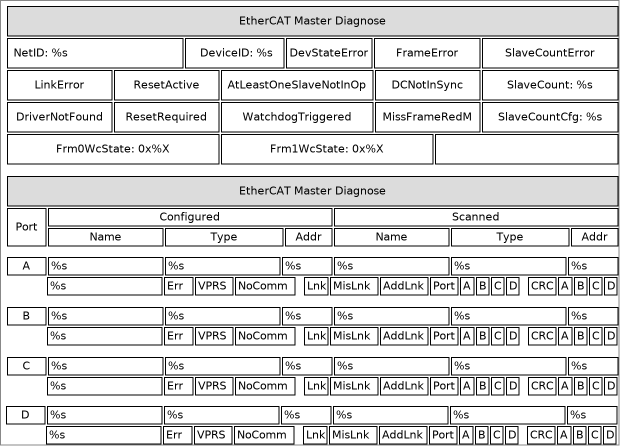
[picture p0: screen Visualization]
VISUALIZATION Visualization  // 620x446
    Rectangle (7,6 611x30), "EtherCAT Master Diagnose"
    Rectangle (7,38 176x30), "NetID: %s", text variable: MAIN.sEcMasterNetId
    Rectangle (185,38 99x30), "DeviceID: %s", text variable: MAIN.nEcMasterDeviceId
    Rectangle (286,38 86x30), "DevStateError", colour toggle: MAIN.bMasterDevStateError
    Rectangle (374,38 106x30), "FrameError", colour toggle: MAIN.bFrameWcStateError
    Rectangle (482,38 136x30), "SlaveCountError", colour toggle: MAIN.bSlaveCountError
    Rectangle (7,70 105x30), "LinkError", colour toggle: MAIN.stMasterDevState.bLinkError
    Rectangle (114,70 105x30), "ResetActive", colour toggle: MAIN.stMasterDevState.bResetActive
    Rectangle (114,102 105x30), "ResetRequired", colour toggle: MAIN.stMasterDevState.bResetRequired
    Rectangle (7,102 105x30), "DriverNotFound", colour toggle: MAIN.stMasterDevState.bDriverNotFound
    Rectangle (221,70 152x30), "AtLeastOneSlaveNotInOp", colour toggle: MAIN.stMasterDevState.bAtLeastOneNotInOp
    Rectangle (221,102 152x30), "WatchdogTriggered", colour toggle: MAIN.stMasterDevState.bWatchdogTriggerd
    Rectangle (375,70 105x30), "DCNotInSync", colour toggle: MAIN.stMasterDevState.bDcNotInSync
    Rectangle (375,102 105x30), "MissFrameRedM", colour toggle: MAIN.stMasterDevState.bMissFrmRedMode
    Rectangle (482,70 136x30), "SlaveCount: %s", text variable: MAIN.nEcMasterSlaveCount, colour toggle: MAIN.bSlaveCountError
    Rectangle (482,102 136x30), "SlaveCountCfg: %s", text variable: MAIN.nEcMasterSlaveCountCfg, colour toggle: MAIN.bSlaveCountError
    Rectangle (7,134 212x30), "Frm0WcState: 0x%X", text variable: FAST.wFrmXWcState, colour toggle: NOT FAST.bFrameWcStateOK
    Rectangle (221,134 212x30), "Frm1WcState: 0x%X", text variable: MAIN.wFrmXWcState, colour toggle: NOT MAIN.bFrameWcStateOK
    Rectangle (435,134 183x30)
    Rectangle (7,176 611x30), "EtherCAT Master Diagnose"
    Rectangle (7,208 39x38), "Port"
    Rectangle (48,208 284x18), "Configured"
    Rectangle (334,208 284x18), "Scanned"
    Rectangle (48,228 115x18), "Name"
    Rectangle (165,228 118x18), "Type"
    Rectangle (285,228 47x18), "Addr"
    Rectangle (451,228 118x18), "Type"
    Rectangle (334,228 115x18), "Name"
    Rectangle (571,228 47x18), "Addr"
    Rectangle (7,257 39x18), "A", invisible if: NOT MAIN.arrDiagSlaveInfo[0].bDiagData
    Rectangle (48,257 115x18), "%s", text variable: MAIN.arrDiagSlaveInfo[0].sName, colour toggle: MAIN.arrDiagSlaveInfoScanned[0].bDifferentName, invisible if: NOT MAIN.arrDiagSlaveInfo[0].bDiagData
    Rectangle (334,257 115x18), "%s", text variable: MAIN.arrDiagSlaveInfoScanned[0].sName, colour toggle: MAIN.arrDiagSlaveInfoScanned[0].bDifferentName, invisible if: NOT MAIN.arrDiagSlaveInfo[0].bDiagData
    Rectangle (165,257 115x18), "%s", text variable: MAIN.arrDiagSlaveInfo[0].sType, colour toggle: MAIN.arrDiagSlaveInfoScanned[0].bDifferentType, invisible if: NOT MAIN.arrDiagSlaveInfo[0].bDiagData
    Rectangle (451,257 115x18), "%s", text variable: MAIN.arrDiagSlaveInfoScanned[0].sType, colour toggle: MAIN.arrDiagSlaveInfoScanned[0].bDifferentType, invisible if: NOT MAIN.arrDiagSlaveInfo[0].bDiagData
    Rectangle (282,257 50x18), "%s", text variable: MAIN.arrDiagSlaveInfo[0].nECAddr, colour toggle: MAIN.arrDiagSlaveInfoScanned[0].bDifferentAddr, invisible if: NOT MAIN.arrDiagSlaveInfo[0].bDiagData
    Rectangle (568,257 50x18), "%s", text variable: MAIN.arrDiagSlaveInfoScanned[0].nECAddr, colour toggle: MAIN.arrDiagSlaveInfoScanned[0].bDifferentAddr, invisible if: NOT MAIN.arrDiagSlaveInfo[0].bDiagData
    Rectangle (47,277 115x18), "%s", text variable: MAIN.arrDiagSlaveInfo[0].stState.eEcState, colour toggle: MAIN.arrDiagSlaveInfo[0].stState.eEcState <> 8, invisible if: NOT MAIN.arrDiagSlaveInfo[0].bDiagData
    Rectangle (164,277 29x18), "Err", colour toggle: MAIN.arrDiagSlaveInfo[0].stState.bError, invisible if: NOT MAIN.arrDiagSlaveInfo[0].bDiagData
    Rectangle (195,277 38x18), "VPRS", colour toggle: MAIN.arrDiagSlaveInfo[0].stState.bInvalidVPRS, invisible if: NOT MAIN.arrDiagSlaveInfo[0].bDiagData
    Rectangle (235,277 60x18), "NoComm", colour toggle: MAIN.arrDiagSlaveInfo[0].stState.bNoCommToSlave, invisible if: NOT MAIN.arrDiagSlaveInfo[0].bDiagData
    Rectangle (304,277 24x18), "Lnk", colour toggle: MAIN.arrDiagSlaveInfo[0].stState.bLinkError, invisible if: NOT MAIN.arrDiagSlaveInfo[0].bDiagData
    Rectangle (330,277 48x18), "MisLnk", colour toggle: MAIN.arrDiagSlaveInfo[0].stState.bMissingLink, invisible if: NOT MAIN.arrDiagSlaveInfo[0].bDiagData
    Rectangle (380,277 48x18), "AddLnk", colour toggle: MAIN.arrDiagSlaveInfo[0].stState.bUnexpectedLink, invisible if: NOT MAIN.arrDiagSlaveInfo[0].bDiagData
    Rectangle (430,277 28x18), "Port", invisible if: NOT MAIN.arrDiagSlaveInfo[0].bDiagData
    Rectangle (460,277 14x18), "A", colour toggle: MAIN.arrDiagSlaveInfo[0].stState.bPortA, invisible if: NOT MAIN.arrDiagSlaveInfo[0].bDiagData
    Rectangle (476,277 13x18), "B", colour toggle: MAIN.arrDiagSlaveInfo[0].stState.bPortB, invisible if: NOT MAIN.arrDiagSlaveInfo[0].bDiagData
    Rectangle (491,277 13x18), "C", colour toggle: MAIN.arrDiagSlaveInfo[0].stState.bPortC, invisible if: NOT MAIN.arrDiagSlaveInfo[0].bDiagData
    Rectangle (506,277 13x18), "D", colour toggle: MAIN.arrDiagSlaveInfo[0].stState.bPortD, invisible if: NOT MAIN.arrDiagSlaveInfo[0].bDiagData
    Rectangle (528,277 28x18), "CRC", colour toggle: MAIN.arrDiagSlaveInfo[0].nSumCRCErrors <> 0, invisible if: NOT MAIN.arrDiagSlaveInfo[0].bDiagData
    Rectangle (558,277 14x18), "A", colour toggle: MAIN.arrDiagSlaveInfo[0].stPortCRCErrors.portA <> 0, invisible if: NOT MAIN.arrDiagSlaveInfo[0].bDiagData
    Rectangle (574,277 13x18), "B", colour toggle: MAIN.arrDiagSlaveInfo[0].stPortCRCErrors.portB <> 0, invisible if: NOT MAIN.arrDiagSlaveInfo[0].bDiagData
    Rectangle (589,277 13x18), "C", colour toggle: MAIN.arrDiagSlaveInfo[0].stPortCRCErrors.portC <> 0, invisible if: NOT MAIN.arrDiagSlaveInfo[0].bDiagData
    Rectangle (604,277 13x18), "D", colour toggle: MAIN.arrDiagSlaveInfo[0].stPortCRCErrors.portD <> 0, invisible if: NOT MAIN.arrDiagSlaveInfo[0].bDiagData
    Rectangle (7,307 39x18), "B", invisible if: MAIN.fbEtherCATDiag.iDiagIndex[1]=0
    Rectangle (48,307 115x18), "%s", text variable: MAIN.arrDiagSlaveInfo[1].sName, colour toggle: MAIN.arrDiagSlaveInfoScanned[1].bDifferentName, invisible if: MAIN.fbEtherCATDiag.iDiagIndex[1]=0
    Rectangle (334,307 115x18), "%s", text variable: MAIN.arrDiagSlaveInfoScanned[1].sName, colour toggle: MAIN.arrDiagSlaveInfoScanned[1].bDifferentName, invisible if: MAIN.fbEtherCATDiag.iDiagIndex[1]=0
    Rectangle (165,307 115x18), "%s", text variable: MAIN.arrDiagSlaveInfo[1].sType, colour toggle: MAIN.arrDiagSlaveInfoScanned[1].bDifferentType, invisible if: MAIN.fbEtherCATDiag.iDiagIndex[1]=0
    Rectangle (451,307 115x18), "%s", text variable: MAIN.arrDiagSlaveInfoScanned[1].sType, colour toggle: MAIN.arrDiagSlaveInfoScanned[1].bDifferentType, invisible if: MAIN.fbEtherCATDiag.iDiagIndex[1]=0
    Rectangle (282,307 50x18), "%s", text variable: MAIN.arrDiagSlaveInfo[1].nECAddr, colour toggle: MAIN.arrDiagSlaveInfoScanned[1].bDifferentAddr, invisible if: MAIN.fbEtherCATDiag.iDiagIndex[1]=0
    Rectangle (568,307 50x18), "%s", text variable: MAIN.arrDiagSlaveInfoScanned[1].nECAddr, colour toggle: MAIN.arrDiagSlaveInfoScanned[1].bDifferentAddr, invisible if: MAIN.fbEtherCATDiag.iDiagIndex[1]=0
    Rectangle (47,327 115x18), "%s", text variable: MAIN.arrDiagSlaveInfo[1].stState.eEcState, colour toggle: MAIN.arrDiagSlaveInfo[1].stState.eEcState <> 8, invisible if: MAIN.fbEtherCATDiag.iDiagIndex[1]=0
    Rectangle (164,327 29x18), "Err", colour toggle: MAIN.arrDiagSlaveInfo[1].stState.bError, invisible if: MAIN.fbEtherCATDiag.iDiagIndex[1]=0
    Rectangle (195,327 38x18), "VPRS", colour toggle: MAIN.arrDiagSlaveInfo[1].stState.bInvalidVPRS, invisible if: MAIN.fbEtherCATDiag.iDiagIndex[1]=0
    Rectangle (235,327 60x18), "NoComm", colour toggle: MAIN.arrDiagSlaveInfo[1].stState.bNoCommToSlave, invisible if: MAIN.fbEtherCATDiag.iDiagIndex[1]=0
    Rectangle (304,327 24x18), "Lnk", colour toggle: MAIN.arrDiagSlaveInfo[1].stState.bLinkError, invisible if: MAIN.fbEtherCATDiag.iDiagIndex[1]=0
    Rectangle (330,327 48x18), "MisLnk", colour toggle: MAIN.arrDiagSlaveInfo[1].stState.bMissingLink, invisible if: MAIN.fbEtherCATDiag.iDiagIndex[1]=0
    Rectangle (380,327 48x18), "AddLnk", colour toggle: MAIN.arrDiagSlaveInfo[1].stState.bUnexpectedLink, invisible if: MAIN.fbEtherCATDiag.iDiagIndex[1]=0
    Rectangle (430,327 28x18), "Port", invisible if: MAIN.fbEtherCATDiag.iDiagIndex[1]=0
    Rectangle (460,327 14x18), "A", colour toggle: MAIN.arrDiagSlaveInfo[1].stState.bPortA, invisible if: MAIN.fbEtherCATDiag.iDiagIndex[1]=0
    Rectangle (476,327 13x18), "B", colour toggle: MAIN.arrDiagSlaveInfo[1].stState.bPortB, invisible if: MAIN.fbEtherCATDiag.iDiagIndex[1]=0
    Rectangle (491,327 13x18), "C", colour toggle: MAIN.arrDiagSlaveInfo[1].stState.bPortC, invisible if: MAIN.fbEtherCATDiag.iDiagIndex[1]=0
    Rectangle (506,327 13x18), "D", colour toggle: MAIN.arrDiagSlaveInfo[1].stState.bPortD, invisible if: MAIN.fbEtherCATDiag.iDiagIndex[1]=0
    Rectangle (528,327 28x18), "CRC", colour toggle: MAIN.arrDiagSlaveInfo[1].nSumCRCErrors <> 0, invisible if: MAIN.fbEtherCATDiag.iDiagIndex[1]=0
    Rectangle (558,327 14x18), "A", colour toggle: MAIN.arrDiagSlaveInfo[1].stPortCRCErrors.portA <> 0, invisible if: MAIN.fbEtherCATDiag.iDiagIndex[1]=0
    Rectangle (574,327 13x18), "B", colour toggle: MAIN.arrDiagSlaveInfo[1].stPortCRCErrors.portB <> 0, invisible if: MAIN.fbEtherCATDiag.iDiagIndex[1]=0
    Rectangle (589,327 13x18), "C", colour toggle: MAIN.arrDiagSlaveInfo[1].stPortCRCErrors.portC <> 0, invisible if: MAIN.fbEtherCATDiag.iDiagIndex[1]=0
    Rectangle (604,327 13x18), "D", colour toggle: MAIN.arrDiagSlaveInfo[1].stPortCRCErrors.portD <> 0, invisible if: MAIN.fbEtherCATDiag.iDiagIndex[1]=0
    Rectangle (7,357 39x18), "C", invisible if: MAIN.fbEtherCATDiag.iDiagIndex[2]=0
    Rectangle (48,357 115x18), "%s", text variable: MAIN.arrDiagSlaveInfo[2].sName, colour toggle: MAIN.arrDiagSlaveInfoScanned[2].bDifferentName, invisible if: MAIN.fbEtherCATDiag.iDiagIndex[2]=0
    Rectangle (334,357 115x18), "%s", text variable: MAIN.arrDiagSlaveInfo[2].sName, colour toggle: MAIN.arrDiagSlaveInfoScanned[2].bDifferentName, invisible if: MAIN.fbEtherCATDiag.iDiagIndex[2]=0
    Rectangle (165,357 115x18), "%s", text variable: MAIN.arrDiagSlaveInfo[2].sType, colour toggle: MAIN.arrDiagSlaveInfoScanned[2].bDifferentType, invisible if: MAIN.fbEtherCATDiag.iDiagIndex[2]=0
    Rectangle (451,357 115x18), "%s", text variable: MAIN.arrDiagSlaveInfoScanned[2].sType, colour toggle: MAIN.arrDiagSlaveInfoScanned[2].bDifferentType, invisible if: MAIN.fbEtherCATDiag.iDiagIndex[2]=0
    Rectangle (282,357 50x18), "%s", text variable: MAIN.arrDiagSlaveInfo[2].nECAddr, colour toggle: MAIN.arrDiagSlaveInfoScanned[2].bDifferentAddr, invisible if: MAIN.fbEtherCATDiag.iDiagIndex[2]=0
    Rectangle (568,357 50x18), "%s", text variable: MAIN.arrDiagSlaveInfoScanned[2].nECAddr, colour toggle: MAIN.arrDiagSlaveInfoScanned[2].bDifferentAddr, invisible if: MAIN.fbEtherCATDiag.iDiagIndex[2]=0
    Rectangle (47,377 115x18), "%s", text variable: MAIN.arrDiagSlaveInfo[2].stState.eEcState, colour toggle: MAIN.arrDiagSlaveInfo[2].stState.eEcState <> 8, invisible if: MAIN.fbEtherCATDiag.iDiagIndex[2]=0
    Rectangle (164,377 29x18), "Err", colour toggle: MAIN.arrDiagSlaveInfo[2].stState.bError, invisible if: MAIN.fbEtherCATDiag.iDiagIndex[2]=0
    Rectangle (195,377 38x18), "VPRS", colour toggle: MAIN.arrDiagSlaveInfo[2].stState.bInvalidVPRS, invisible if: MAIN.fbEtherCATDiag.iDiagIndex[2]=0
    Rectangle (235,377 60x18), "NoComm", colour toggle: MAIN.arrDiagSlaveInfo[2].stState.bNoCommToSlave, invisible if: MAIN.fbEtherCATDiag.iDiagIndex[2]=0
    Rectangle (304,377 24x18), "Lnk", colour toggle: MAIN.arrDiagSlaveInfo[2].stState.bLinkError, invisible if: MAIN.fbEtherCATDiag.iDiagIndex[2]=0
    Rectangle (330,377 48x18), "MisLnk", colour toggle: MAIN.arrDiagSlaveInfo[2].stState.bMissingLink, invisible if: MAIN.fbEtherCATDiag.iDiagIndex[2]=0
    Rectangle (380,377 48x18), "AddLnk", colour toggle: MAIN.arrDiagSlaveInfo[2].stState.bUnexpectedLink, invisible if: MAIN.fbEtherCATDiag.iDiagIndex[2]=0
    Rectangle (430,377 28x18), "Port", invisible if: MAIN.fbEtherCATDiag.iDiagIndex[2]=0
    Rectangle (460,377 14x18), "A", colour toggle: MAIN.arrDiagSlaveInfo[2].stState.bPortA, invisible if: MAIN.fbEtherCATDiag.iDiagIndex[2]=0
    Rectangle (476,377 13x18), "B", colour toggle: MAIN.arrDiagSlaveInfo[2].stState.bPortB, invisible if: MAIN.fbEtherCATDiag.iDiagIndex[2]=0
    Rectangle (491,377 13x18), "C", colour toggle: MAIN.arrDiagSlaveInfo[2].stState.bPortC, invisible if: MAIN.fbEtherCATDiag.iDiagIndex[2]=0
    Rectangle (506,377 13x18), "D", colour toggle: MAIN.arrDiagSlaveInfo[2].stState.bPortD, invisible if: MAIN.fbEtherCATDiag.iDiagIndex[2]=0
    Rectangle (528,377 28x18), "CRC", colour toggle: MAIN.arrDiagSlaveInfo[2].nSumCRCErrors <> 0, invisible if: MAIN.fbEtherCATDiag.iDiagIndex[2]=0
    Rectangle (558,377 14x18), "A", colour toggle: MAIN.arrDiagSlaveInfo[2].stPortCRCErrors.portA <> 0, invisible if: MAIN.fbEtherCATDiag.iDiagIndex[2]=0
    Rectangle (574,377 13x18), "B", colour toggle: MAIN.arrDiagSlaveInfo[2].stPortCRCErrors.portB <> 0, invisible if: MAIN.fbEtherCATDiag.iDiagIndex[2]=0
    Rectangle (589,377 13x18), "C", colour toggle: MAIN.arrDiagSlaveInfo[2].stPortCRCErrors.portC <> 0, invisible if: MAIN.fbEtherCATDiag.iDiagIndex[2]=0
    Rectangle (604,377 13x18), "D", colour toggle: MAIN.arrDiagSlaveInfo[2].stPortCRCErrors.portD <> 0, invisible if: MAIN.fbEtherCATDiag.iDiagIndex[2]=0
    Rectangle (6,406 39x18), "D", invisible if: MAIN.fbEtherCATDiag.iDiagIndex[3]=0
    Rectangle (47,406 115x18), "%s", text variable: MAIN.arrDiagSlaveInfo[3].sName, colour toggle: MAIN.arrDiagSlaveInfoScanned[3].bDifferentName, invisible if: MAIN.fbEtherCATDiag.iDiagIndex[3]=0
    Rectangle (333,406 115x18), "%s", text variable: MAIN.arrDiagSlaveInfoScanned[3].sName, colour toggle: MAIN.arrDiagSlaveInfoScanned[3].bDifferentName, invisible if: MAIN.fbEtherCATDiag.iDiagIndex[3]=0
    Rectangle (164,406 115x18), "%s", text variable: MAIN.arrDiagSlaveInfo[3].sType, colour toggle: MAIN.arrDiagSlaveInfoScanned[3].bDifferentType, invisible if: MAIN.fbEtherCATDiag.iDiagIndex[3]=0
    Rectangle (450,406 115x18), "%s", text variable: MAIN.arrDiagSlaveInfoScanned[3].sType, colour toggle: MAIN.arrDiagSlaveInfoScanned[3].bDifferentType, invisible if: MAIN.fbEtherCATDiag.iDiagIndex[3]=0
    Rectangle (281,406 50x18), "%s", text variable: MAIN.arrDiagSlaveInfo[3].nECAddr, colour toggle: MAIN.arrDiagSlaveInfoScanned[3].bDifferentAddr, invisible if: MAIN.fbEtherCATDiag.iDiagIndex[3]=0
    Rectangle (567,406 50x18), "%s", text variable: MAIN.arrDiagSlaveInfoScanned[3].nECAddr, colour toggle: MAIN.arrDiagSlaveInfoScanned[3].bDifferentAddr, invisible if: MAIN.fbEtherCATDiag.iDiagIndex[3]=0
    Rectangle (46,426 115x18), "%s", text variable: MAIN.arrDiagSlaveInfo[3].stState.eEcState, colour toggle: MAIN.arrDiagSlaveInfo[3].stState.eEcState <> 8, invisible if: MAIN.fbEtherCATDiag.iDiagIndex[3]=0
    Rectangle (163,426 29x18), "Err", colour toggle: MAIN.arrDiagSlaveInfo[3].stState.bError, invisible if: MAIN.fbEtherCATDiag.iDiagIndex[3]=0
    Rectangle (194,426 38x18), "VPRS", colour toggle: MAIN.arrDiagSlaveInfo[3].stState.bInvalidVPRS, invisible if: MAIN.fbEtherCATDiag.iDiagIndex[3]=0
    Rectangle (234,426 60x18), "NoComm", colour toggle: MAIN.arrDiagSlaveInfo[3].stState.bNoCommToSlave, invisible if: MAIN.fbEtherCATDiag.iDiagIndex[3]=0
    Rectangle (303,426 24x18), "Lnk", colour toggle: MAIN.arrDiagSlaveInfo[3].stState.bLinkError, invisible if: MAIN.fbEtherCATDiag.iDiagIndex[3]=0
    Rectangle (329,426 48x18), "MisLnk", colour toggle: MAIN.arrDiagSlaveInfo[3].stState.bMissingLink, invisible if: MAIN.fbEtherCATDiag.iDiagIndex[3]=0
    Rectangle (379,426 48x18), "AddLnk", colour toggle: MAIN.arrDiagSlaveInfo[3].stState.bUnexpectedLink, invisible if: MAIN.fbEtherCATDiag.iDiagIndex[3]=0
    Rectangle (429,426 28x18), "Port", invisible if: MAIN.fbEtherCATDiag.iDiagIndex[3]=0
    Rectangle (459,426 14x18), "A", colour toggle: MAIN.arrDiagSlaveInfo[3].stState.bPortA, invisible if: MAIN.fbEtherCATDiag.iDiagIndex[3]=0
    Rectangle (475,426 13x18), "B", colour toggle: MAIN.arrDiagSlaveInfo[3].stState.bPortB, invisible if: MAIN.fbEtherCATDiag.iDiagIndex[3]=0
    Rectangle (490,426 13x18), "C", colour toggle: MAIN.arrDiagSlaveInfo[3].stState.bPortC, invisible if: MAIN.fbEtherCATDiag.iDiagIndex[3]=0
    Rectangle (505,426 13x18), "D", colour toggle: MAIN.arrDiagSlaveInfo[3].stState.bPortD, invisible if: MAIN.fbEtherCATDiag.iDiagIndex[3]=0
    Rectangle (527,426 28x18), "CRC", colour toggle: MAIN.arrDiagSlaveInfo[3].nSumCRCErrors <> 0, invisible if: MAIN.fbEtherCATDiag.iDiagIndex[3]=0
    Rectangle (557,426 14x18), "A", colour toggle: MAIN.arrDiagSlaveInfo[3].stPortCRCErrors.portA <> 0, invisible if: MAIN.fbEtherCATDiag.iDiagIndex[3]=0
    Rectangle (573,426 13x18), "B", colour toggle: MAIN.arrDiagSlaveInfo[3].stPortCRCErrors.portB <> 0, invisible if: MAIN.fbEtherCATDiag.iDiagIndex[3]=0
    Rectangle (588,426 13x18), "C", colour toggle: MAIN.arrDiagSlaveInfo[3].stPortCRCErrors.portC <> 0, invisible if: MAIN.fbEtherCATDiag.iDiagIndex[3]=0
    Rectangle (603,426 13x18), "D", colour toggle: MAIN.arrDiagSlaveInfo[3].stPortCRCErrors.portD <> 0, invisible if: MAIN.fbEtherCATDiag.iDiagIndex[3]=0
END_VISUALIZATION
